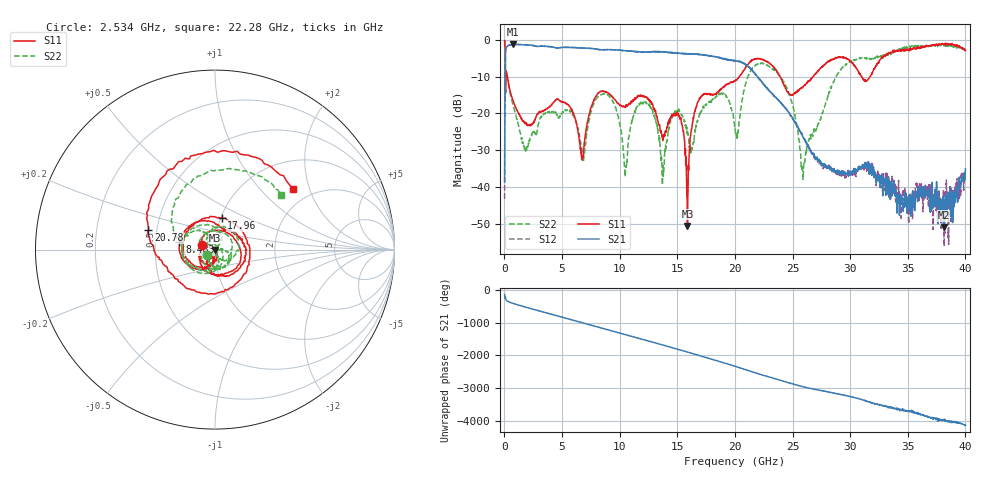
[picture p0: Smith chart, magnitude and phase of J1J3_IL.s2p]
!Agilent Technologies,N5230A,US43500312,A.07.50.67
!Agilent N5230A: A.07.50.67
!Date: Thursday, March 05, 2015 11:19:29
!Correction: S11(Full 2 Port(1,2))
!S21(Full 2 Port(1,2))
!S12(Full 2 Port(1,2))
!S22(Full 2 Port(1,2))
!S2P File: Measurements: S11, S21, S12, S22:
# Hz S  dB  R 50
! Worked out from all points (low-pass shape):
!   1601 points, 10 MHz to 40 GHz, reference 50 ohm
!   highest |S21| = -1.19 dB at 759.8 MHz (marker M1); lowest = -51.1 dB at 38.1 GHz (marker M2)
!   |S21| within 3 dB of the highest: 83.11 MHz to 17.43 GHz (17.35 GHz wide, 198 % of centre); 17.43 GHz to 17.57 GHz (135.2 MHz wide, 0.772 % of centre)
!   lowest |S11| = -50.7 dB at 15.88 GHz (marker M3), VSWR 1.01, Z = 49.9 - j0.273 ohm
!   |S11| at or under -10 dB: 248 MHz to 20.39 GHz (20.14 GHz wide, 195 % of centre); 23.92 GHz to 26.75 GHz (2.832 GHz wide, 11.2 % of centre); 30.99 GHz to 31.72 GHz (735.3 MHz wide, 2.34 % of centre)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
!   |S22| runs from -39.5 to -0.1 dB; largest |S21 - S12| = 0.015
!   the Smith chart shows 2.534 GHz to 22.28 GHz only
!   S11 on the Smith chart (normalised r, x): 2.534 GHz: 0.87, +0.04; 8.483 GHz: 0.67, +0.06; 17.96 GHz: 1.01, +0.37; 20.78 GHz: 0.45, +0.12; 22.28 GHz: 1.60, +1.56
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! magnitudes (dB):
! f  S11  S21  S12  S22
! 10 MHz  -0.2  -38.7  -43.2  -0.1
! 259.9 MHz  -10.3  -1.7  -1.7  -10.5
! 759.8 MHz  -16.6  -1.2  -1.2  -17.8
! 2.534 GHz  -22.4  -1.5  -1.5  -25.0
! 5.384 GHz  -17.3  -2.0  -2.0  -19.2
! 6.683 GHz  -31.8  -2.2  -2.2  -29.3
! 8.483 GHz  -13.9  -2.7  -2.7  -14.8
! 10.48 GHz  -18.1  -2.9  -2.9  -36.4
! 11.68 GHz  -15.1  -3.2  -3.3  -17.4
! 13.36 GHz  -22.7  -3.1  -3.2  -25.5
! 15.16 GHz  -20.8  -3.6  -3.6  -19.1
! 15.88 GHz  -50.7  -3.8  -3.7  -24.6
! 17.96 GHz  -14.9  -4.4  -4.4  -16.9
! 20 GHz  -11.1  -5.6  -5.7  -23.5
! 20.78 GHz  -8.2  -6.3  -6.4  -13.8
! 22.28 GHz  -5.2  -11.2  -11.3  -6.4
! 24.58 GHz  -14.1  -19.3  -19.4  -13.7
! 25.88 GHz  -13.0  -26.4  -26.0  -36.4
! 26.68 GHz  -10.4  -30.8  -31.0  -25.7
! 33.35 GHz  -3.6  -39.0  -43.0  -3.8
! 38.1 GHz  -1.2  -51.1  -40.8  -1.5
! 40 GHz  -2.9  -35.1  -35.7  -2.4
